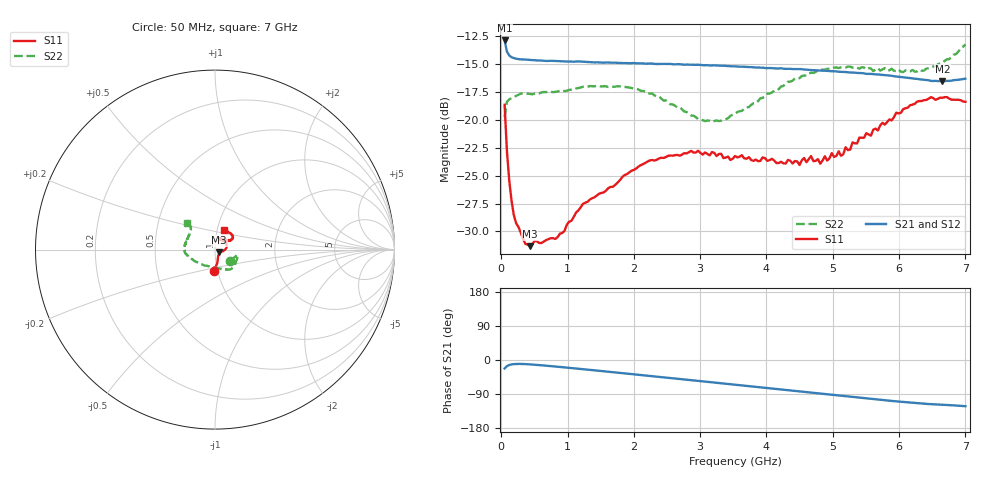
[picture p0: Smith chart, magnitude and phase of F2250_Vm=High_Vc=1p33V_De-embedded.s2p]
! Integrated Device Technology
! Corporate Headquarters
! 6024 Silver Creek Valley Road
! San Jose, CA 95138  USA
! Phone:  1-408-284-8200
! Toll Free:  1-800-223-1366
! Webpage:  http://www.idt.com/
! Timing and RF Division
! 515 Groton Road, Suite 102
! Westford, MA 01886-6024
! Device:  F2250
! Description: Voltage Variable RF Attenuator
! Frequency:  50.0 -  6000.00 MHz
! Package:  3x3 mm Thin QFN Plastic Package: 16 pin
! Ports:  2 RF, 3 DC
!  Pin  1  = GND
!  Pin  2  = NC
!  Pin  3  = RF1  = Port 1
!  Pin  4  = NC
!  Pin  5  = GND
!  Pin  6  = GND
!  Pin  7  = GND
!  Pin  8  = GND
!  Pin  9  = NC
!  Pin 10  = RF2  = Port 2
!  Pin 11  = NC
!  Pin 12  = GND
!  Pin 13  = GND
!  Pin 14  = VCNTRL
!  Pin 15  = VDD
!  Pin 16  = VMODE
! Vcntrl:  1.330 Volts
! Vmode:  +3.300 Volts
! Vdd:  +3.30  Volts
! Current:  1.331 mA
! Data:  The device was measured on a the F2250 evaluation board which has
!  individual transmission lines to the RF pins.  Data was collected
!  using a calibrated network analyzer.  The evaluation board was
!  de-embedded using a TRL calibration technique.
!  The reference plane is the edge of the package pin.
! Misc:  SN 10
!  Action Tracker AT0258
! Date Measured:  2014-11-26
! Date:  2015-10-15  MJV
! Note:
!  Integrated Device Technology supplies this data as a sample of measured
!  data at the package pin for this product.  Your particular data for this
!  product may vary.
!  Data was taken at 25 degrees C.
!  Integrated Device Technology reserves the right to change this data at anytime.
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# GHz S dB R 50
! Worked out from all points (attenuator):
!   201 points, 50 MHz to 7 GHz, reference 50 ohm
!   highest |S21| = -12.89 dB at 50 MHz (marker M1); lowest = -16.5 dB at 6.652 GHz (marker M2)
!   lowest |S11| = -31.3 dB at 432.2 MHz (marker M3), VSWR 1.06, Z = 52.3 - j1.54 ohm
!   |S11| at or under -10 dB: start of sweep to end of sweep
!   |S22| runs from -20.2 to -13.2 dB; largest |S21 - S12| = 0.00075
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0.05  -18.65 -91.8  -12.89 -22.3  -12.89 -22.3  -19.76 -37.0
0.08475  -22.79 -79.1  -13.88 -16.2  -13.88 -16.2  -18.39 -19.0
0.1195  -25.40 -72.9  -14.23 -13.2  -14.24 -13.2  -18.16 -14.1
0.189  -28.54 -59.7  -14.47 -10.8  -14.46 -10.8  -17.93 -12.5
0.36275  -31.10 -35.7  -14.60 -10.8  -14.61 -10.8  -17.68 -14.2
0.43225  -31.32 -32.9  -14.63 -11.5  -14.64 -11.5  -17.68 -15.4
0.84925  -30.51 -18.0  -14.74 -17.8  -14.71 -17.8  -17.46 -28.5
1.2315  -27.53 -13.3  -14.80 -24.2  -14.81 -24.2  -17.03 -38.1
1.857  -24.96 0.5  -14.91 -35.1  -14.92 -35.1  -17.04 -50.3
2.37825  -23.46 13.9  -14.99 -44.4  -14.98 -44.4  -17.90 -62.0
3.07325  -22.92 35.8  -15.10 -57.0  -15.09 -57.1  -20.12 -94.4
3.525  -23.24 51.5  -15.21 -65.3  -15.22 -65.3  -19.47 -125.1
4.7065  -23.70 63.3  -15.55 -86.9  -15.56 -86.9  -15.80 -170.8
5.08875  -22.82 50.5  -15.69 -93.9  -15.69 -93.9  -15.36 -179.3
5.1235  -23.22 50.7  -15.70 -94.5  -15.70 -94.5  -15.29 179.8
5.193  -22.46 45.9  -15.72 -95.7  -15.72 -95.8  -15.30 178.6
5.2625  -22.66 42.1  -15.76 -96.9  -15.74 -97.0  -15.23 177.5
5.29725  -22.03 41.6  -15.76 -97.6  -15.75 -97.7  -15.32 176.5
5.85325  -19.96 31.9  -16.03 -107.4  -16.03 -107.5  -15.56 162.0
6.27025  -18.37 33.5  -16.33 -114.0  -16.33 -114.0  -15.67 148.9
6.6525  -18.03 43.7  -16.54 -118.2  -16.52 -118.3  -14.88 137.8
7  -18.38 64.0  -16.31 -121.9  -16.31 -122.1  -13.25 136.5
